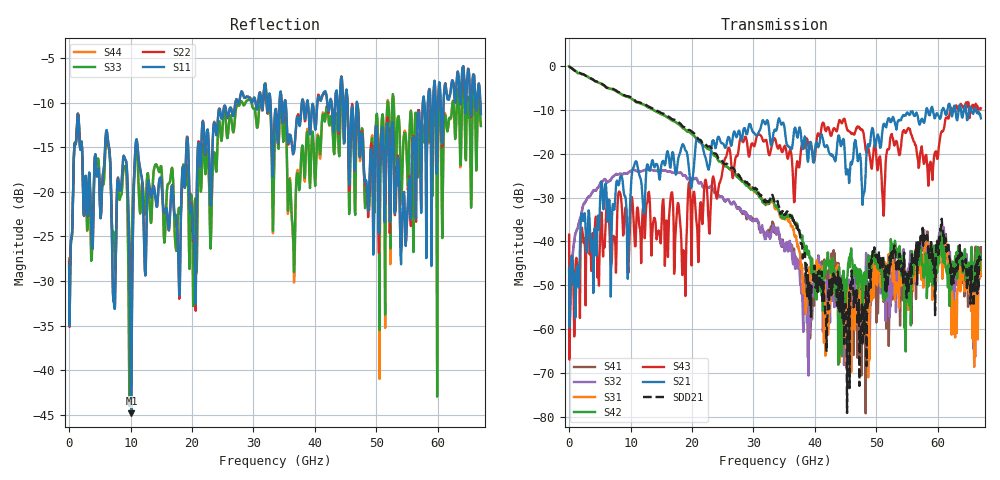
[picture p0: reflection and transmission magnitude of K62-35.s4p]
!Agilent Technologies,N5247A,US50470101,A.10.25.02
!Agilent N5247A: A.10.25.02
!Date: Tuesday, May 12, 2015 13:42:13
!Correction: Sdd11(Full 4 Port(1,2,3,4))
!Sdc11(Full 4 Port(1,2,3,4))
!Sdd12(Full 4 Port(1,2,3,4))
!Sdc12(Full 4 Port(1,2,3,4))
!Scd11(Full 4 Port(1,2,3,4))
!Scc11(Full 4 Port(1,2,3,4))
!Scd12(Full 4 Port(1,2,3,4))
!Scc12(Full 4 Port(1,2,3,4))
!Sdd21(Full 4 Port(1,2,3,4))
!Sdc21(Full 4 Port(1,2,3,4))
!Sdd22(Full 4 Port(1,2,3,4))
!Sdc22(Full 4 Port(1,2,3,4))
!Scd21(Full 4 Port(1,2,3,4))
!Scc21(Full 4 Port(1,2,3,4))
!Scd22(Full 4 Port(1,2,3,4))
!Scc22(Full 4 Port(1,2,3,4))
!Balanced Topology: BBAL
!S4P File: Measurements: <Sdd11,Sdc11,Sdd12,Sdc12>,
!<Scd11,Scc11,Scd12,Scc12>,
!<Sdd21,Sdc21,Sdd22,Sdc22>,
!<Scd21,Scc21,Scd22,Scc22>:
# Hz S  dB  R 50
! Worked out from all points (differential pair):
!   801 points, 10 MHz to 67 GHz, reference 50 ohm
!   strongest paths, dB at 10 MHz, 16.76 GHz, 33.51 GHz, 50.25 GHz, 67 GHz:
!     S21: -46.1, -20.0, -14.5, -15.6, -11.9
!     S43: -38.5, -28.8, -16.6, -23.5, -9.6
!     S42: -0.1, -12.4, -31.8, -45.9, -44.0
!     S31: 0.0, -12.4, -32.5, -46.8, -47.6
!     S32: -48.5, -24.3, -37.7, -46.4, -45.8
!     S41: -46.7, -24.3, -36.9, -56.4, -41.3
!   taken as a pair (ports 2,1 in; 4,3 out), SDD21 dB: 0.0, -12.1, -31.3, -45.0, -44.0
!   lowest |S11| = -44.9 dB at 10.14 GHz (marker M1), VSWR 1.01, Z = 49.4 + j0.0377 ohm
!   |S11| at or under -10 dB: start of sweep to 27.06 GHz; 35.23 GHz to 37.88 GHz (2.648 GHz wide, 7.24 % of centre); 46.89 GHz to 57.56 GHz (10.67 GHz wide, 20.4 % of centre)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
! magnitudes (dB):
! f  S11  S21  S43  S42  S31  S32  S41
! 10 MHz  -28.3  -46.1  -38.5  -0.1  0.0  -48.5  -46.7
! 6.207 GHz  -13.4  -32.7  -30.2  -5.0  -5.0  -26.6  -26.6
! 10.14 GHz  -44.9  -25.8  -30.2  -7.4  -7.4  -23.8  -23.9
! 18.68 GHz  -18.3  -18.2  -42.2  -14.3  -14.3  -25.0  -25.0
! 41.71 GHz  -8.7  -18.5  -14.7  -47.5  -66.0  -52.7  -45.1
! 51.09 GHz  -14.2  -13.6  -32.2  -53.0  -48.8  -48.3  -46.6
! 67 GHz  -11.3  -11.9  -9.6  -44.0  -47.6  -45.8  -41.3
